(* Logix 5000 Rung export; software revision 16.04; part 2 of 2 *)
(* AOI69EAFC, continued *)

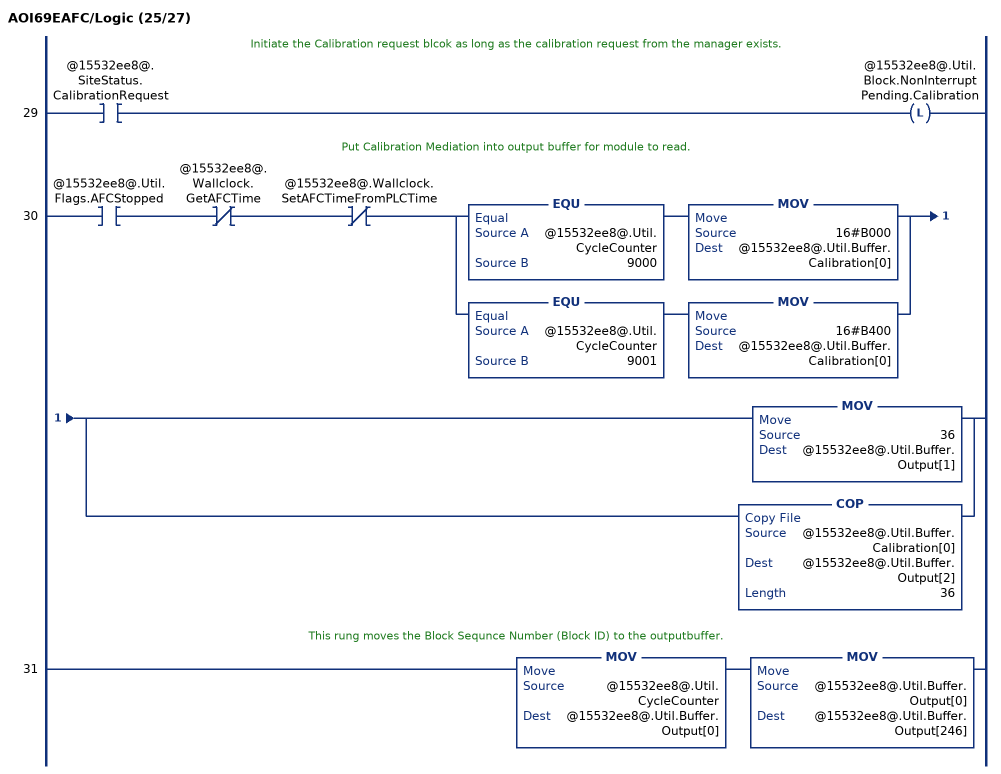
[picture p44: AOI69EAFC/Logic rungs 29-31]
   // Initiate the Calibration request blcok as long as the calibration request from the manager exists.
   29: XIC(@15532ee8@.SiteStatus.CalibrationRequest)OTL(@15532ee8@.Util.Block.NonInterruptPending.Calibration);
   // Put Calibration Mediation into output buffer for module to read.
   30: XIC(@15532ee8@.Util.Flags.AFCStopped)XIO(@15532ee8@.Wallclock.GetAFCTime)XIO(@15532ee8@.Wallclock.SetAFCTimeFromPLCTime)[EQU(@15532ee8@.Util.CycleCounter,9000) MOV(16#B000,@15532ee8@.Util.Buffer.Calibration[0]) ,EQU(@15532ee8@.Util.CycleCounter,9001) MOV(16#B400,@15532ee8@.Util.Buffer.Calibration[0]) ][MOV(36,@15532ee8@.Util.Buffer.Output[1]) ,COP(@15532ee8@.Util.Buffer.Calibration[0],@15532ee8@.Util.Buffer.Output[2],36) ];
   // This rung moves the Block Sequnce Number (Block ID) to the outputbuffer.
   31: MOV(@15532ee8@.Util.CycleCounter,@15532ee8@.Util.Buffer.Output[0])MOV(@15532ee8@.Util.Buffer.Output[0],@15532ee8@.Util.Buffer.Output[246]);
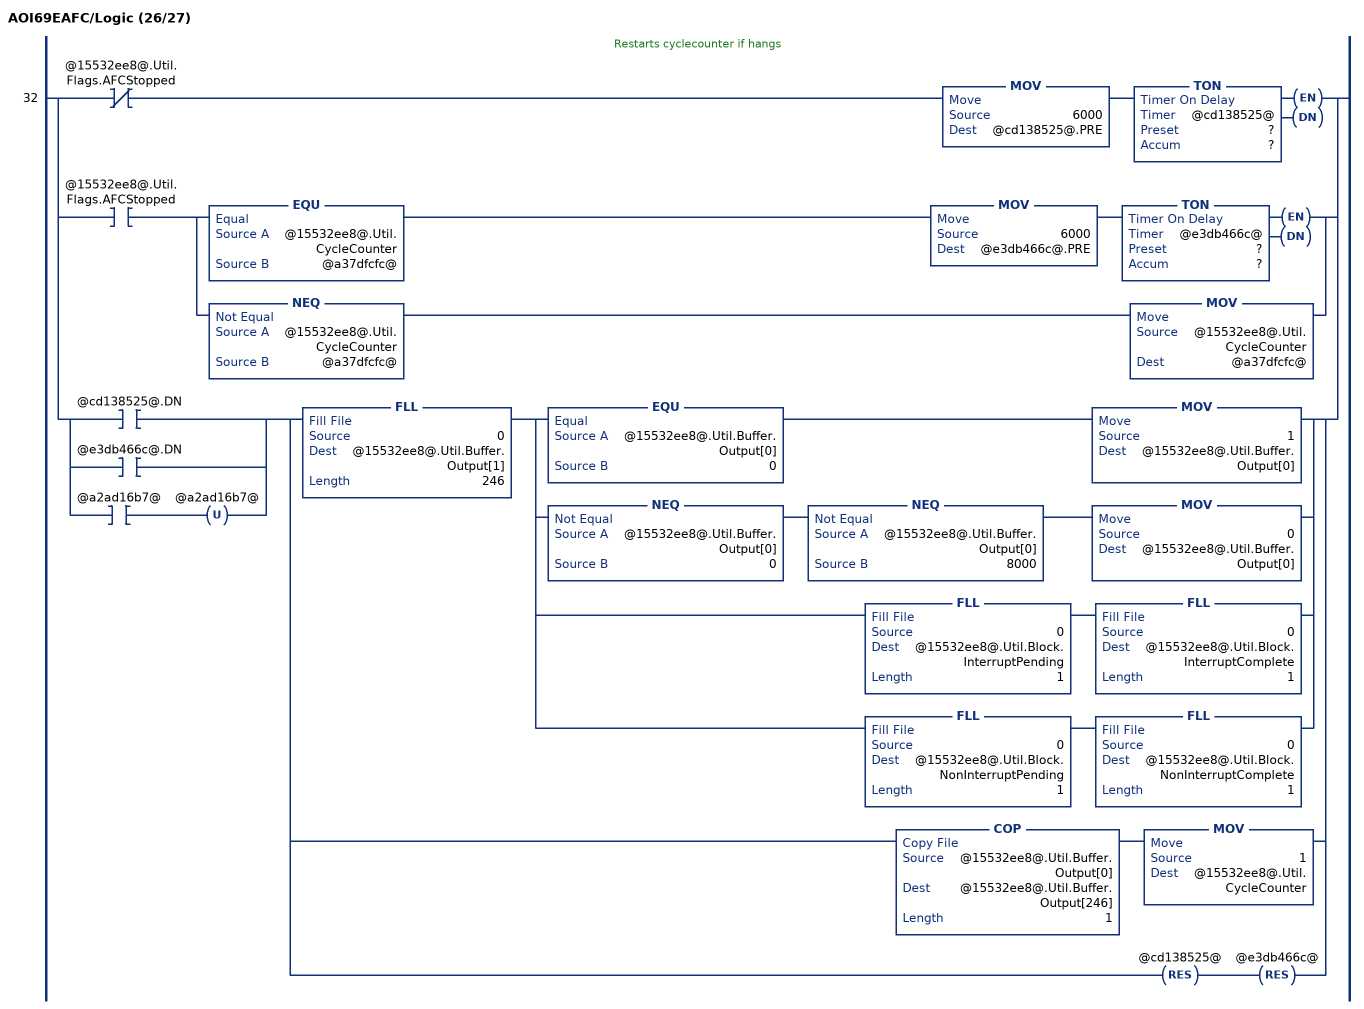
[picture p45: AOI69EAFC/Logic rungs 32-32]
   // Restarts cyclecounter if hangs
   32: [XIO(@15532ee8@.Util.Flags.AFCStopped) MOV(6000,@cd138525@.PRE) TON(@cd138525@,?,?) ,XIC(@15532ee8@.Util.Flags.AFCStopped) [EQU(@15532ee8@.Util.CycleCounter,@a37dfcfc@) MOV(6000,@e3db466c@.PRE) TON(@e3db466c@,?,?) ,NEQ(@15532ee8@.Util.CycleCounter,@a37dfcfc@) MOV(@15532ee8@.Util.CycleCounter,@a37dfcfc@) ] ,[[XIC(@cd138525@.DN) ,XIC(@e3db466c@.DN) ] ,XIC(@a2ad16b7@) OTU(@a2ad16b7@) ] [FLL(0,@15532ee8@.Util.Buffer.Output[1],246) [EQU(@15532ee8@.Util.Buffer.Output[0],0) MOV(1,@15532ee8@.Util.Buffer.Output[0]) ,NEQ(@15532ee8@.Util.Buffer.Output[0],0) NEQ(@15532ee8@.Util.Buffer.Output[0],8000) MOV(0,@15532ee8@.Util.Buffer.Output[0]) ,FLL(0,@15532ee8@.Util.Block.InterruptPending,1) FLL(0,@15532ee8@.Util.Block.InterruptComplete,1) ,FLL(0,@15532ee8@.Util.Block.NonInterruptPending,1) FLL(0,@15532ee8@.Util.Block.NonInterruptComplete,1) ] ,COP(@15532ee8@.Util.Buffer.Output[0],@15532ee8@.Util.Buffer.Output[246],1) MOV(1,@15532ee8@.Util.CycleCounter) ,RES(@cd138525@) RES(@e3db466c@) ] ];
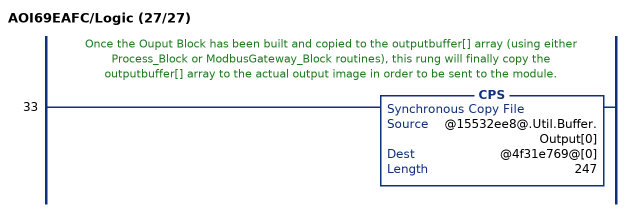
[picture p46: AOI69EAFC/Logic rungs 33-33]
   // Once the Ouput Block has been built and copied to the outputbuffer[] array (using either Process_Block or ModbusGateway_Block routines), this rung will finally copy the outputbuffer[] array to the actual output image in order to be sent to the module.
   33: CPS(@15532ee8@.Util.Buffer.Output[0],@4f31e769@[0],247);
END_ROUTINE

ROUTINE Prescan   (* ladder *)
// Prescan
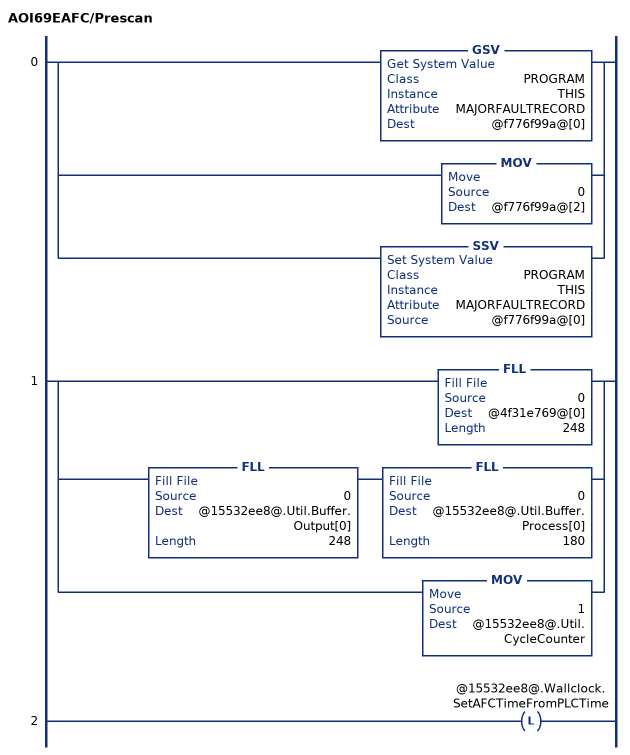
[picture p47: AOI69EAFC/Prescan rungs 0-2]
   0: [GSV(PROGRAM,THIS,MAJORFAULTRECORD,@f776f99a@[0]) ,MOV(0,@f776f99a@[2]) ,SSV(PROGRAM,THIS,MAJORFAULTRECORD,@f776f99a@[0]) ];
   1: [FLL(0,@4f31e769@[0],248) ,FLL(0,@15532ee8@.Util.Buffer.Output[0],248) FLL(0,@15532ee8@.Util.Buffer.Process[0],180) ,MOV(1,@15532ee8@.Util.CycleCounter) ];
   2: OTL(@15532ee8@.Wallclock.SetAFCTimeFromPLCTime);
END_ROUTINE
END_ADD_ON_INSTRUCTION

VAR_GLOBAL   (* controller tags *)
   Local:1:I : AB:1756_MODULE_INT_496Bytes:I:0;
   AFC : AFCEModuleDef;
   Local:1:O : AB:1756_MODULE_INT_494Bytes:O:0;
   AOI69EAFC : AOI69EAFC;
END_VAR

PROGRAM MainProgram

ROUTINE MainRoutine   (* ladder *)
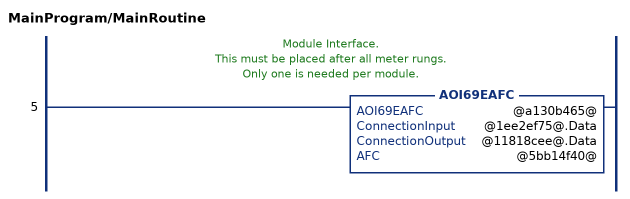
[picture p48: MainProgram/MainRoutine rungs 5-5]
   // Module Interface.
   // This must be placed after all meter rungs.
   // Only one is needed per module.
   5: AOI69EAFC(@a130b465@,@1ee2ef75@.Data,@11818cee@.Data,@5bb14f40@);
END_ROUTINE
END_PROGRAM
